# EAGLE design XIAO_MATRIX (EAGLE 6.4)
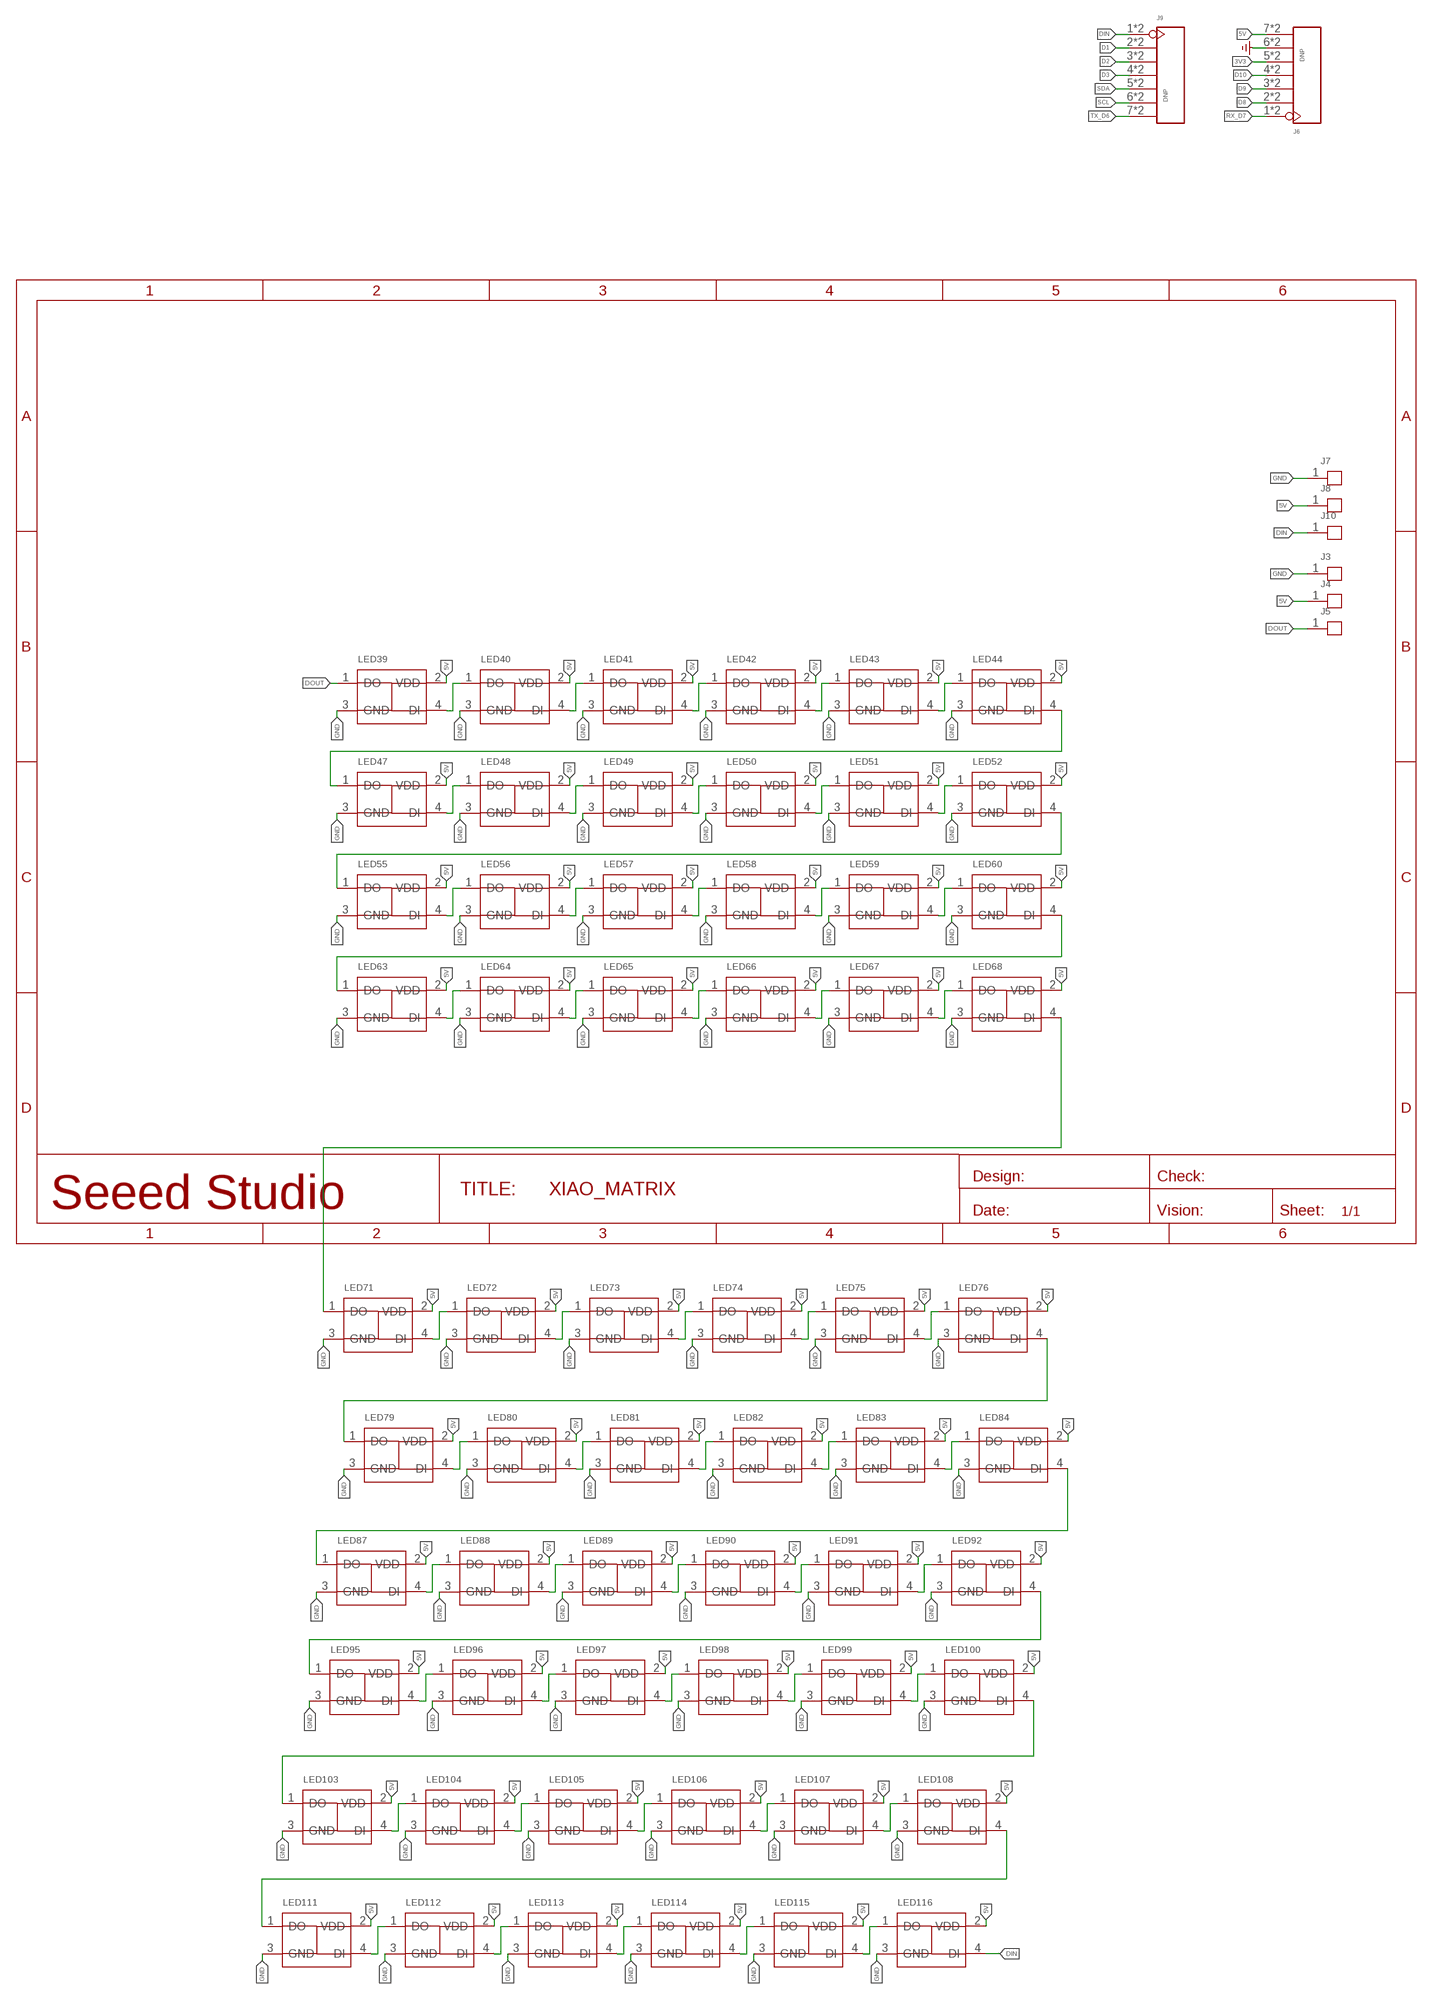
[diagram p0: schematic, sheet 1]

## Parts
J3  HEADER-1P-1.5MM  [H1P-3.5/1.5MM]
J4  HEADER-1P-1.5MM  [H1P-3.5/1.5MM]
J5  HEADER-1P-1.5MM  [H1P-3.5/1.5MM]
J6  DNP  HEADER-7P-HALF-HOLE-2.54  [H7-HALF-HOLE-2.54]
J7  HEADER-1P-1.5MM  [H1P-3.5/1.5MM]
J8  HEADER-1P-1.5MM  [H1P-3.5/1.5MM]
J9  DNP  HEADER-7P-HALF-HOLE-2.54  [H7-HALF-HOLE-2.54]
J10  HEADER-1P-1.5MM  [H1P-3.5/1.5MM]
LED39  LED-1010  [LED-1010]
LED40  LED-1010  [LED-1010]
LED41  LED-1010  [LED-1010]
LED42  LED-1010  [LED-1010]
LED43  LED-1010  [LED-1010]
LED44  LED-1010  [LED-1010]
LED47  LED-1010  [LED-1010]
LED48  LED-1010  [LED-1010]
LED49  LED-1010  [LED-1010]
LED50  LED-1010  [LED-1010]
LED51  LED-1010  [LED-1010]
LED52  LED-1010  [LED-1010]
LED55  LED-1010  [LED-1010]
LED56  LED-1010  [LED-1010]
LED57  LED-1010  [LED-1010]
LED58  LED-1010  [LED-1010]
LED59  LED-1010  [LED-1010]
LED60  LED-1010  [LED-1010]
LED63  LED-1010  [LED-1010]
LED64  LED-1010  [LED-1010]
LED65  LED-1010  [LED-1010]
LED66  LED-1010  [LED-1010]
LED67  LED-1010  [LED-1010]
LED68  LED-1010  [LED-1010]
LED71  LED-1010  [LED-1010]
LED72  LED-1010  [LED-1010]
LED73  LED-1010  [LED-1010]
LED74  LED-1010  [LED-1010]
LED75  LED-1010  [LED-1010]
LED76  LED-1010  [LED-1010]
LED79  LED-1010  [LED-1010]
LED80  LED-1010  [LED-1010]
LED81  LED-1010  [LED-1010]
LED82  LED-1010  [LED-1010]
LED83  LED-1010  [LED-1010]
LED84  LED-1010  [LED-1010]
LED87  LED-1010  [LED-1010]
LED88  LED-1010  [LED-1010]
LED89  LED-1010  [LED-1010]
LED90  LED-1010  [LED-1010]
LED91  LED-1010  [LED-1010]
LED92  LED-1010  [LED-1010]
LED95  LED-1010  [LED-1010]
LED96  LED-1010  [LED-1010]
LED97  LED-1010  [LED-1010]
LED98  LED-1010  [LED-1010]
LED99  LED-1010  [LED-1010]
LED100  LED-1010  [LED-1010]
LED103  LED-1010  [LED-1010]
LED104  LED-1010  [LED-1010]
LED105  LED-1010  [LED-1010]
LED106  LED-1010  [LED-1010]
LED107  LED-1010  [LED-1010]
LED108  LED-1010  [LED-1010]
LED111  LED-1010  [LED-1010]
LED112  LED-1010  [LED-1010]
LED113  LED-1010  [LED-1010]
LED114  LED-1010  [LED-1010]
LED115  LED-1010  [LED-1010]
LED116  LED-1010  [LED-1010]

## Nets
3V3: J6.5 J6.17
5V: J4.1 J6.7 J6.19 J8.1 LED39.2(VDD) LED40.2(VDD) LED41.2(VDD) LED42.2(VDD) LED43.2(VDD) LED44.2(VDD) LED47.2(VDD) LED48.2(VDD) LED49.2(VDD) LED50.2(VDD) LED51.2(VDD) LED52.2(VDD) LED55.2(VDD) LED56.2(VDD) LED57.2(VDD) LED58.2(VDD) LED59.2(VDD) LED60.2(VDD) LED63.2(VDD) LED64.2(VDD) LED65.2(VDD) LED66.2(VDD) LED67.2(VDD) LED68.2(VDD) LED71.2(VDD) LED72.2(VDD) LED73.2(VDD) LED74.2(VDD) LED75.2(VDD) LED76.2(VDD) LED79.2(VDD) LED80.2(VDD) LED81.2(VDD) LED82.2(VDD) LED83.2(VDD) LED84.2(VDD) LED87.2(VDD) LED88.2(VDD) LED89.2(VDD) LED90.2(VDD) LED91.2(VDD) LED92.2(VDD) LED95.2(VDD) LED96.2(VDD) LED97.2(VDD) LED98.2(VDD) LED99.2(VDD) LED100.2(VDD) LED103.2(VDD) LED104.2(VDD) LED105.2(VDD) LED106.2(VDD) LED107.2(VDD) LED108.2(VDD) LED111.2(VDD) LED112.2(VDD) LED113.2(VDD) LED114.2(VDD) LED115.2(VDD) LED116.2(VDD)
D1: J9.2 J9.14
D2: J9.3 J9.15
D3: J9.4 J9.16
D8: J6.2 J6.14
D9: J6.3 J6.15
D10: J6.4 J6.16
DIN: J9.1 J9.13 J10.1 LED116.4(DI)
DOUT: J5.1 LED39.1(DO)
GND: J3.1 J6.6 J6.18 J7.1 LED39.3(GND) LED40.3(GND) LED41.3(GND) LED42.3(GND) LED43.3(GND) LED44.3(GND) LED47.3(GND) LED48.3(GND) LED49.3(GND) LED50.3(GND) LED51.3(GND) LED52.3(GND) LED55.3(GND) LED56.3(GND) LED57.3(GND) LED58.3(GND) LED59.3(GND) LED60.3(GND) LED63.3(GND) LED64.3(GND) LED65.3(GND) LED66.3(GND) LED67.3(GND) LED68.3(GND) LED71.3(GND) LED72.3(GND) LED73.3(GND) LED74.3(GND) LED75.3(GND) LED76.3(GND) LED79.3(GND) LED80.3(GND) LED81.3(GND) LED82.3(GND) LED83.3(GND) LED84.3(GND) LED87.3(GND) LED88.3(GND) LED89.3(GND) LED90.3(GND) LED91.3(GND) LED92.3(GND) LED95.3(GND) LED96.3(GND) LED97.3(GND) LED98.3(GND) LED99.3(GND) LED100.3(GND) LED103.3(GND) LED104.3(GND) LED105.3(GND) LED106.3(GND) LED107.3(GND) LED108.3(GND) LED111.3(GND) LED112.3(GND) LED113.3(GND) LED114.3(GND) LED115.3(GND) LED116.3(GND) ; supply symbol labelled GND_POWER
N$24: LED39.4(DI) LED40.1(DO)
N$25: LED40.4(DI) LED41.1(DO)
N$26: LED41.4(DI) LED42.1(DO)
N$27: LED42.4(DI) LED43.1(DO)
N$28: LED43.4(DI) LED44.1(DO)
N$31: LED47.4(DI) LED48.1(DO)
N$32: LED48.4(DI) LED49.1(DO)
N$33: LED49.4(DI) LED50.1(DO)
N$34: LED50.4(DI) LED51.1(DO)
N$35: LED51.4(DI) LED52.1(DO)
N$38: LED55.4(DI) LED56.1(DO)
N$39: LED56.4(DI) LED57.1(DO)
N$40: LED57.4(DI) LED58.1(DO)
N$41: LED58.4(DI) LED59.1(DO)
N$42: LED59.4(DI) LED60.1(DO)
N$45: LED63.4(DI) LED64.1(DO)
N$46: LED64.4(DI) LED65.1(DO)
N$47: LED65.4(DI) LED66.1(DO)
N$48: LED66.4(DI) LED67.1(DO)
N$49: LED67.4(DI) LED68.1(DO)
N$52: LED71.4(DI) LED72.1(DO)
N$53: LED72.4(DI) LED73.1(DO)
N$54: LED73.4(DI) LED74.1(DO)
N$55: LED74.4(DI) LED75.1(DO)
N$56: LED75.4(DI) LED76.1(DO)
N$59: LED79.4(DI) LED80.1(DO)
N$60: LED80.4(DI) LED81.1(DO)
N$61: LED81.4(DI) LED82.1(DO)
N$62: LED82.4(DI) LED83.1(DO)
N$63: LED83.4(DI) LED84.1(DO)
N$66: LED87.4(DI) LED88.1(DO)
N$67: LED88.4(DI) LED89.1(DO)
N$68: LED89.4(DI) LED90.1(DO)
N$69: LED90.4(DI) LED91.1(DO)
N$70: LED91.4(DI) LED92.1(DO)
N$73: LED95.4(DI) LED96.1(DO)
N$74: LED96.4(DI) LED97.1(DO)
N$75: LED97.4(DI) LED98.1(DO)
N$76: LED98.4(DI) LED99.1(DO)
N$77: LED99.4(DI) LED100.1(DO)
N$80: LED103.4(DI) LED104.1(DO)
N$81: LED104.4(DI) LED105.1(DO)
N$82: LED105.4(DI) LED106.1(DO)
N$83: LED106.4(DI) LED107.1(DO)
N$84: LED107.4(DI) LED108.1(DO)
N$87: LED111.4(DI) LED112.1(DO)
N$88: LED112.4(DI) LED113.1(DO)
N$89: LED113.4(DI) LED114.1(DO)
N$90: LED114.4(DI) LED115.1(DO)
N$91: LED115.4(DI) LED116.1(DO)
N$95: LED44.4(DI) LED47.1(DO)
N$96: LED52.4(DI) LED55.1(DO)
N$97: LED60.4(DI) LED63.1(DO)
N$98: LED68.4(DI) LED71.1(DO)
N$99: LED76.4(DI) LED79.1(DO)
N$100: LED84.4(DI) LED87.1(DO)
N$101: LED92.4(DI) LED95.1(DO)
N$102: LED100.4(DI) LED103.1(DO)
N$103: LED108.4(DI) LED111.1(DO)
RX_D7: J6.1 J6.13
SCL: J9.6 J9.18
SDA: J9.5 J9.17
TX_D6: J9.7 J9.19

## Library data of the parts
J3-J5 J7 J8 J10 = Connector-new:HEADER-1P
J6 J9 = Connector-new_2:HEADER-7P-HALF-HOLE
LED39-LED44 LED47-LED52 LED55-LED60 LED63-LED68 LED71-LED76 LED79-LED84 LED87-LED92 LED95-LED100 LED103-LED108 LED111-LED116 = 0703:LED-1010

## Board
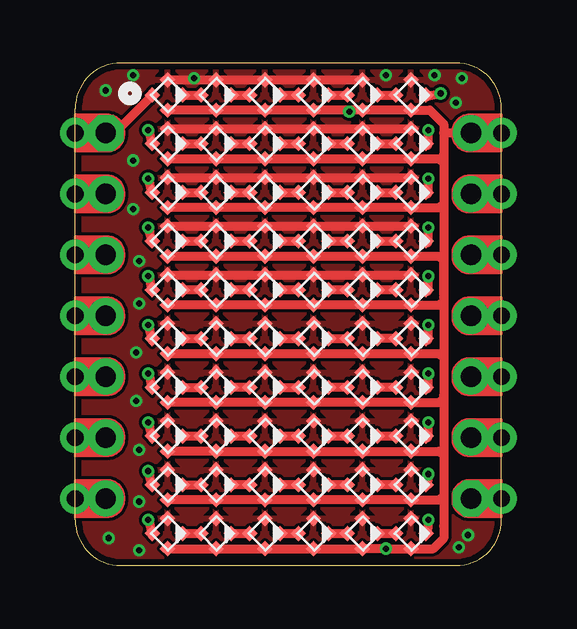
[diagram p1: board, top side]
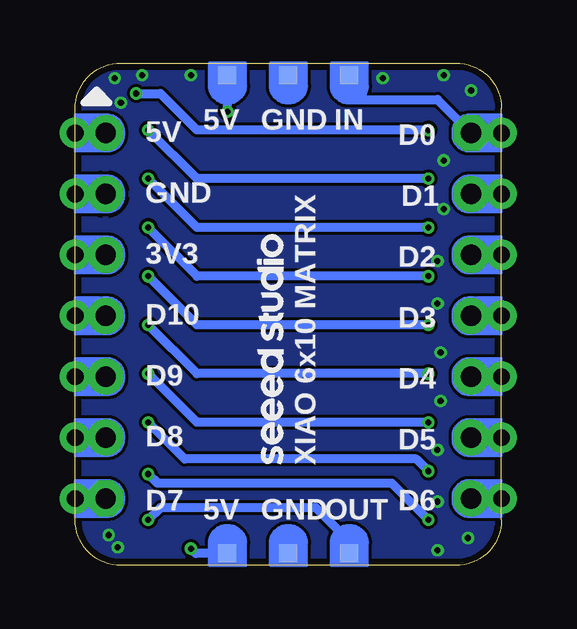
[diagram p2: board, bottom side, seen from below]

Size 17.78 x 20.95 mm. Coordinates in mm from the lower left corner, seen from the top.
Outline: 15.88,20.95 1.91,20.95 arc90 0,19.05 0,1.91 arc90 1.91,0 15.88,0 arc90 17.78,1.91 17.78,19.05 arc90 15.88,20.95
Copper layers (1*16): Top 0.035mm / dielectric 1.5mm / Bottom 0.035mm
Design rules "SeeedStudio_2layer_DRU_no_angle_20140221 *": minimum track width 1mil, minimum drill 10mil, track to track 5mil, track to pad 5mil, pad to pad 5mil, via to via 5mil, smd to smd 0mil, copper to edge 10mil, drill to drill 10mil, minimum pad ring 4mil, minimum via ring 4mil, stop-mask expansion 2mil, vias tented up to drill 25mil, thermal gap 10mil

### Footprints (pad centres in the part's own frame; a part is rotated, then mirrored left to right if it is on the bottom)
H1P-3.5/1.5MM = smd 0.762 x 0.762 bottom: 1 0,0.127
H7-HALF-HOLE-2.54 = drill 0.85 pad 1.5 octagon: 1 0,7.62 | drill 0.85 pad 1.5: 2 0,5.08; 3 0,2.54; 4 0,0; 5 0,-2.54; 6 0,-5.08; 7 0,-7.62 | drill 0.7 pad 1.27: 13 -1.27,7.62; 14 -1.27,5.08; 15 -1.27,2.54; 16 -1.27,0; 17 -1.27,-2.54; 18 -1.27,-5.08; 19 -1.27,-7.62
LED-1010 = smd 0.45 x 0.45: 1 -0.425,0.425; 2 0.464,0.425; 3 -0.425,-0.464; 4 0.464,-0.464

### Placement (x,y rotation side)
J3  8.89,0.38 0 top
J4  11.43,0.38 0 top
J5  6.35,0.38 0 top
J6  16.51,10.41 180 top
J7  8.89,20.57 180 top
J8  11.43,20.57 180 top
J9  1.27,10.41 0 top
J10  6.35,20.57 180 top
LED39  14.03,1.33 225 top
LED40  12,1.33 225 top
LED41  9.97,1.33 225 top
LED42  7.94,1.33 225 top
LED43  5.91,1.33 225 top
LED44  3.87,1.33 225 top
LED47  14.03,3.37 225 top
LED48  12,3.37 225 top
LED49  9.97,3.37 225 top
LED50  7.94,3.37 225 top
LED51  5.91,3.37 225 top
LED52  3.87,3.37 225 top
LED55  14.03,5.4 225 top
LED56  12,5.4 225 top
LED57  9.97,5.4 225 top
LED58  7.94,5.4 225 top
LED59  5.91,5.4 225 top
LED60  3.87,5.4 225 top
LED63  14.03,7.43 225 top
LED64  12,7.43 225 top
LED65  9.97,7.43 225 top
LED66  7.94,7.43 225 top
LED67  5.91,7.43 225 top
LED68  3.87,7.43 225 top
LED71  14.03,9.46 225 top
LED72  12,9.46 225 top
LED73  9.97,9.46 225 top
LED74  7.94,9.46 225 top
LED75  5.91,9.46 225 top
LED76  3.87,9.46 225 top
LED79  14.03,11.49 225 top
LED80  12,11.49 225 top
LED81  9.97,11.49 225 top
LED82  7.94,11.49 225 top
LED83  5.91,11.49 225 top
LED84  3.87,11.49 225 top
LED87  14.03,13.53 225 top
LED88  12,13.53 225 top
LED89  9.97,13.53 225 top
LED90  7.94,13.53 225 top
LED91  5.91,13.53 225 top
LED92  3.87,13.53 225 top
LED95  14.03,15.56 225 top
LED96  12,15.56 225 top
LED97  9.97,15.56 225 top
LED98  7.94,15.56 225 top
LED99  5.91,15.56 225 top
LED100  3.87,15.56 225 top
LED103  14.03,17.59 225 top
LED104  12,17.59 225 top
LED105  9.97,17.59 225 top
LED106  7.94,17.59 225 top
LED107  5.91,17.59 225 top
LED108  3.87,17.59 225 top
LED111  14.03,19.62 225 top
LED112  12,19.62 225 top
LED113  9.97,19.62 225 top
LED114  7.94,19.62 225 top
LED115  5.91,19.62 225 top
LED116  3.87,19.62 225 top
U$3  [LOGO-SEEED-NEW-1X9.6MM]  9.02,4.19 90 bottom

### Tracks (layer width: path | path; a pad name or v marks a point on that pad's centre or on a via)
3V3
  Top 0.381: J6.17 J6.5
5V  (via drill 0.25 pad 0.51)
  Top 0.152: 15.37,1.65 15.37,2.55 15.18,2.74 | 15.24,4.7 15.37,4.57 | 15.37,6.73 15.24,6.86 15.24,6.98 15.37,7.11 15.37,8.64 15.24,8.76 | 15.24,10.92 15.37,10.79 | 15.24,12.83 15.24,11.3 15.37,11.18 | 15.24,14.99 15.37,14.99 | 15.17,16.96 15.18,16.96 15.37,17.14
  Top 0.381: LED44.2 LED43.2 LED42.2 LED41.2 LED40.2 v12.95,0.71 LED39.2 14.93,0.71 15.37,1.14 15.37,1.65 15.37,4.57 15.37,6.73 15.37,7.11 15.37,10.79 15.37,11.18 15.37,14.99 15.37,17.14 15.37,18.03 | LED52.2 LED51.2 LED50.2 LED49.2 LED48.2 LED47.2 15.18,2.74 15.24,2.79 | LED60.2 LED59.2 LED58.2 LED57.2 LED56.2 LED55.2 15.17,4.77 15.24,4.7 | LED68.2 LED67.2 LED66.2 LED65.2 LED64.2 LED63.2 15.18,6.8 15.24,6.86 | LED76.2 LED75.2 LED74.2 LED73.2 LED72.2 LED71.2 15.17,8.83 15.24,8.76 | LED84.2 LED83.2 LED82.2 LED81.2 LED80.2 LED79.2 15.18,10.87 15.24,10.92 | LED92.2 LED91.2 LED90.2 LED89.2 LED88.2 LED87.2 15.17,12.9 15.24,12.83 | LED100.2 LED99.2 LED98.2 LED97.2 LED96.2 LED95.2 15.18,14.93 15.24,14.99 | LED108.2 LED107.2 LED106.2 LED105.2 LED104.2 LED103.2 15.17,16.96 15.24,16.89 | LED112.2 LED111.2 14.79,18.99 15.37,18.41 15.37,18.03 | LED112.2 LED113.2 LED114.2 LED115.2 LED116.2 | LED112.2 11.5,18.99 v11.43,18.92 | J6.7 15.37,18.03
  Bottom 0.152: J6.7 J6.19
  Bottom 0.381: v11.43,18.92 J8.1 | J4.1 12.76,0.51 v12.95,0.71
D1
  Bottom 0.152: J9.2 J9.14
D2
  Bottom 0.152: J9.3 J9.15
D3
  Bottom 0.152: J9.4 J9.16
D8
  Bottom 0.152: J6.2 J6.14
D9
  Bottom 0.152: J6.3 J6.15
D10
  Bottom 0.152: J6.4 J6.16
DIN
  Top 0.305: 1.78,18.16 1.4,18.16 J9.1
  Top 0.381: LED116.4 3.22,19.6 1.78,18.16
  Bottom 0.152: J9.1 J9.13
  Bottom 0.381: J9.1 2.67,19.43 6.35,19.43 J10.1
DOUT  (via drill 0.25 pad 0.51)
  Top 0.381: v14.73,1.91 14.7,1.4 LED39.1
  Bottom 0.381: J5.1 6.35,1.02 7.75,2.41 14.22,2.41 v14.73,1.91
GND  (via drill 0.25 pad 0.51)
  Top 0.381: LED116.3 LED115.3 LED114.3 LED113.3 LED112.3 | LED108.3 LED107.3 LED106.3 LED105.3 LED104.3 LED103.3 | LED100.3 LED99.3 LED98.3 LED97.3 LED96.3 LED95.3 | LED92.3 LED91.3 LED90.3 LED89.3 LED88.3 LED87.3 | LED84.3 LED83.3 LED82.3 LED81.3 LED80.3 LED79.3
  other vias: 1.27,19.81 16.13,20.32 16.38,1.27 1.4,1.14 2.41,20.45 4.95,20.32 15.88,19.3 14.99,20.45 12.95,20.45 2.41,16.89 2.41,14.86 2.67,12.7 2.67,10.92 2.54,8.89 2.54,6.86 2.67,4.83 2.67,2.67 2.67,0.64 16,0.76
  pour Top (isolate 0.127): 0,-0.13 0,21.08 17.78,21.08 17.78,-0.13
  pour Bottom: 0,-0.13 0,21.08 17.78,21.08 17.78,-0.13
N$24
  Top 0.381: LED40.1 LED39.4
N$25
  Top 0.381: LED41.1 LED40.4
N$26
  Top 0.381: LED42.1 LED41.4
N$27
  Top 0.381: LED43.1 LED42.4
N$28
  Top 0.381: LED44.1 LED43.4
N$31
  Top 0.381: LED47.4 LED48.1
N$32
  Top 0.381: LED48.4 LED49.1
N$33
  Top 0.381: LED49.4 LED50.1
N$34
  Top 0.381: LED50.4 LED51.1
N$35
  Top 0.381: LED52.1 LED51.4
N$38
  Top 0.381: LED56.1 LED55.4
N$39
  Top 0.381: LED57.1 LED56.4
N$40
  Top 0.381: LED58.1 LED57.4
N$41
  Top 0.381: LED59.1 LED58.4
N$42
  Top 0.381: LED60.1 LED59.4
N$45
  Top 0.381: LED63.4 LED64.1
N$46
  Top 0.381: LED64.4 LED65.1
N$47
  Top 0.381: LED66.1 LED65.4
N$48
  Top 0.381: LED66.4 LED67.1
N$49
  Top 0.381: LED68.1 LED67.4
N$52
  Top 0.381: LED71.4 LED72.1
N$53
  Top 0.381: LED73.1 LED72.4
N$54
  Top 0.381: LED74.1 LED73.4
N$55
  Top 0.381: LED75.1 LED74.4
N$56
  Top 0.381: LED76.1 LED75.4
N$59
  Top 0.381: LED79.4 LED80.1
N$60
  Top 0.381: LED80.4 LED81.1
N$61
  Top 0.381: LED81.4 LED82.1
N$62
  Top 0.381: LED82.4 LED83.1
N$63
  Top 0.381: LED83.4 LED84.1
N$66
  Top 0.381: LED88.1 LED87.4
N$67
  Top 0.381: LED89.1 LED88.4
N$68
  Top 0.381: LED90.1 LED89.4
N$69
  Top 0.381: LED91.1 LED90.4
N$70
  Top 0.381: LED92.1 LED91.4
N$73
  Top 0.381: LED96.1 LED95.4
N$74
  Top 0.381: LED97.1 LED96.4
N$75
  Top 0.381: LED98.1 LED97.4
N$76
  Top 0.381: LED99.1 LED98.4
N$77
  Top 0.381: LED100.1 LED99.4
N$80
  Top 0.381: LED104.1 LED103.4
N$81
  Top 0.381: LED105.1 LED104.4
N$82
  Top 0.381: LED106.1 LED105.4
N$83
  Top 0.381: LED107.1 LED106.4
N$84
  Top 0.381: LED108.1 LED107.4
N$87
  Top 0.381: LED112.1 LED111.4
N$88
  Top 0.381: LED113.1 LED112.4
N$89
  Top 0.381: LED114.1 LED113.4
N$90
  Top 0.381: LED115.1 LED114.4
N$91
  Top 0.381: LED116.1 LED115.4
N$95  (via drill 0.25 pad 0.51)
  Top 0.381: LED44.4 3.11,1.84 v3.05,1.91 | v14.73,3.81 14.7,3.43 LED47.1
  Bottom 0.381: v3.05,1.91 4.57,3.43 14.35,3.43 v14.73,3.81
N$96  (via drill 0.25 pad 0.51)
  Top 0.381: LED52.4 3.11,3.75 v3.05,3.94 | v14.73,5.97 14.7,5.33 LED55.1
  Bottom 0.381: v3.05,3.94 3.56,4.45 13.21,4.45 v14.73,5.97
N$97  (via drill 0.25 pad 0.51)
  Top 0.381: LED60.4 3.11,5.78 v3.05,5.97 | v14.73,8 14.7,7.37 LED63.1
  Bottom 0.381: v3.05,5.97 12.7,5.97 v14.73,8
N$98  (via drill 0.25 pad 0.51)
  Top 0.381: LED68.4 3.11,7.94 v3.05,8 | v14.73,10.03 14.7,9.4 LED71.1
  Bottom 0.381: v3.05,8 12.7,8 v14.73,10.03
N$99  (via drill 0.25 pad 0.51)
  Top 0.381: LED76.4 3.11,9.84 v3.05,10.03 | v14.73,12.06 14.7,11.43 LED79.1
  Bottom 0.381: v3.05,10.03 12.7,10.03 v14.73,12.06
N$100  (via drill 0.25 pad 0.51)
  Top 0.381: LED84.4 3.11,12 v3.05,12.06 | v14.73,14.1 14.7,13.46 LED87.1
  Bottom 0.381: v3.05,12.06 12.7,12.06 v14.73,14.1
N$101  (via drill 0.25 pad 0.51)
  Top 0.381: LED92.4 3.11,13.91 v3.05,14.1 | v14.73,16.13 14.7,15.49 LED95.1
  Bottom 0.381: v3.05,14.1 12.7,14.1 v14.73,16.13
N$102  (via drill 0.25 pad 0.51)
  Top 0.381: LED100.4 3.11,15.94 v3.05,16.13 | v14.73,18.16 14.7,17.53 LED103.1
  Bottom 0.381: v3.05,16.13 12.7,16.13 v14.73,18.16
N$103  (via drill 0.25 pad 0.51)
  Top 0.381: LED108.4 3.11,18.1 v3.05,18.16 | v15.24,19.69 14.7,19.56 LED111.1
  Bottom 0.381: v3.05,18.16 12.7,18.16 14.22,19.69 v15.24,19.69
RX_D7
  Bottom 0.152: J6.1 J6.13
SCL
  Bottom 0.152: J9.6 J9.18
SDA
  Bottom 0.152: J9.5 J9.17
TX_D6
  Bottom 0.152: J9.7 J9.19

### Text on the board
bPlace: IN | GND | 5V | D0 | 5V | D1 | GND | D2 | 3V3 | D10 | D3 | D4 | D9 | D8 | D5 | XIAO 6x10 MATRIX | D6 | D7 | OUT | GND | 5V
tTest: CH | B | R
bTest: MTDI | MTDO | VUSB | D0 | EN | D1 | GND | GND | MTMS | MTCK | D2 | BAT | 3V3 | D3 | D10 | D4 | D9 | D5 | D8 | Seeed | D6 | XIAO ESP32C3 | D7 | Booot | RST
